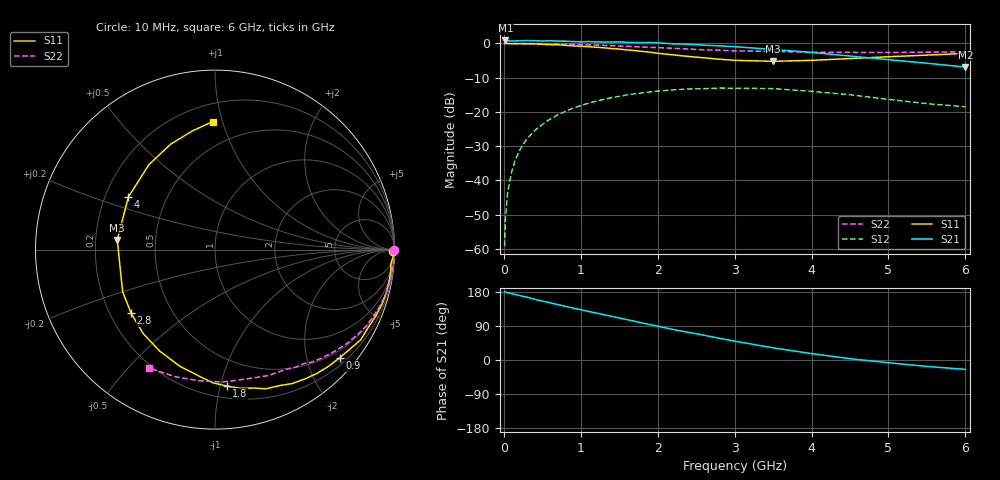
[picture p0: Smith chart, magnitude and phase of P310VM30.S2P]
! SIEMENS Small Signal Semiconductors
! BFP181
! Si NPN RF Bipolar Junction Transistor in SOT143
! VCE = 10 V  IC = 0.3 mA
! Common Emitter S-Parameters:  March  1996
# GHz  S  MA  R  50
!  f  S11  S21  S12  S22
! GHz  MAG  ANG  MAG  ANG  MAG  ANG  MAG  ANG
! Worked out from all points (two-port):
!   36 points, 10 MHz to 6 GHz, reference 50 ohm
!   highest |S21| = 0.84 dB at 20 MHz (marker M1); lowest = -6.9 dB at 6 GHz (marker M2)
!   |S21| within 3 dB of the highest: start of sweep to 3.724 GHz
!   lowest |S11| = -5.2 dB at 3.5 GHz (marker M3), VSWR 3.42, Z = 14.7 + j2.28 ohm
!   |S11| at or under -10 dB: nowhere
!   |S22| runs from -2.7 to 0.0 dB; largest |S21 - S12| = 1.1
!   S11 on the Smith chart (normalised r, x): 10 MHz: open; 900 MHz: 0.34, -2.64; 1.8 GHz: 0.29, -1.05; 2.8 GHz: 0.29, -0.31; 4 GHz: 0.30, +0.26; 6 GHz: 0.32, +0.93
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0.01  0.9904 -0.5  1.083 179.8  0.0011 87.9  0.9994 -0.2
0.02  0.9967 -0.9  1.102 179.8  0.0027 88.9  0.999 -0.4
0.05  0.9937 -2.0  1.095 177.5  0.0068 89.2  0.9983 -1.2
0.1  0.9835 -4.6  1.082 175.3  0.0131 86.1  0.9983 -2.3
0.15  0.9864 -6.8  1.086 172.9  0.0201 84.5  0.9986 -3.5
0.25  0.9859 -11.4  1.092 167.9  0.0335 82.3  0.9956 -5.8
0.4  0.9794 -18.0  1.093 160.3  0.0534 76.7  0.9923 -9.2
0.5  0.9688 -22.7  1.083 155.5  0.0655 72.8  0.9881 -11.5
0.9  0.9195 -41.0  1.063 136.9  0.1136 59.4  0.9656 -20.4
1.1  0.8939 -50.4  1.063 128.2  0.1339 52.9  0.9505 -24.6
1.5  0.8255 -70.0  1.052 111.0  0.1684 40.5  0.9137 -32.7
1.8  0.7627 -85.1  1.025 97.4  0.1894 32.1  0.8856 -38.3
2  0.7175 -95.6  1.019 89.3  0.2013 26.4  0.8668 -41.9
2.2  0.6787 -106.8  0.984 80.5  0.2093 20.8  0.8467 -45.6
2.4  0.6438 -118.6  0.972 73.0  0.216 15.4  0.8271 -49.2
2.8  0.5868 -142.8  0.92 57.4  0.2228 5.6  0.7947 -55.5
3  0.5653 -155.6  0.894 49.8  0.2217 0.6  0.777 -58.9
3.5  0.5472 174.3  0.816 32.2  0.2187 -10.4  0.7622 -67.0
4  0.5647 148.7  0.738 16.9  0.1994 -19.6  0.7419 -76.3
4.5  0.5998 127.8  0.653 3.5  0.1779 -27.1  0.7389 -86.6
5.5  0.6734 100.7  0.513 -17.0  0.1318 -29.3  0.7425 -107.8
6  0.7132 91.0  0.451 -24.7  0.1189 -25.6  0.7553 -119.0
